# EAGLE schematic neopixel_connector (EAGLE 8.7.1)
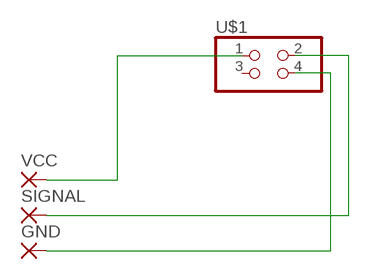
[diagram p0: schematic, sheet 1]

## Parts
GND  SMD2  [SMD1,27-2,54]
SIGNAL  SMD2  [SMD1,27-2,54]
U$1  PINHD-2X2-SMD  [2X02SMD]
VCC  SMD2  [SMD1,27-2,54]

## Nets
N$1: U$1.1 VCC.1(P)
N$2: SIGNAL.1(P) U$1.2
N$3: GND.1(P) U$1.4
Unconnected: U$1.3

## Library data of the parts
GND SIGNAL VCC = wirepad:SMD2: SMD PAD
U$1 = fab:PINHD-2X2-SMD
